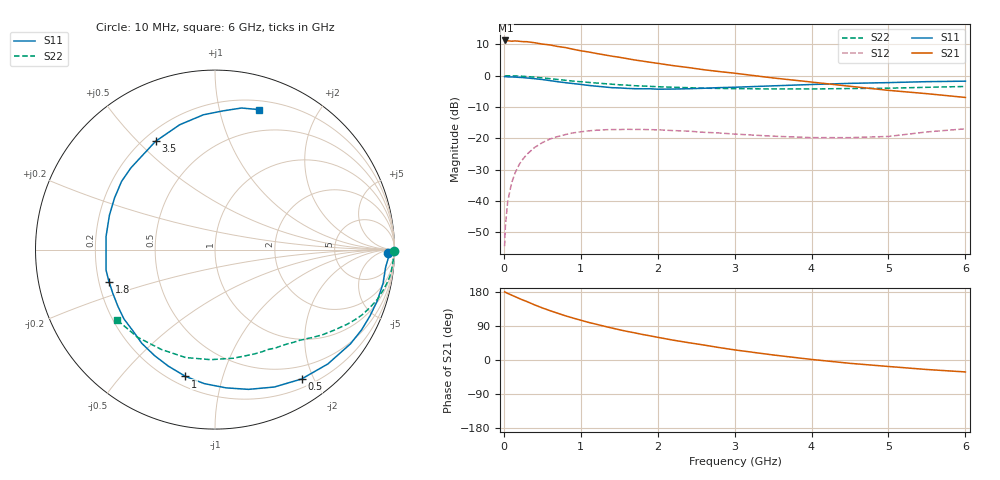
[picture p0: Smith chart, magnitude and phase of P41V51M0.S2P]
! SIEMENS Small Signal Semiconductors
! BFP182
! Si NPN RF Bipolar Junction Transistor in SOT143
! VCE = 1.5 V  IC = 1 mA
! Common Emitter S-Parameters:  March  1996
# GHz  S  MA  R  50
!  f  S11  S21  S12  S22
! GHz  MAG  ANG  MAG  ANG  MAG  ANG  MAG  ANG
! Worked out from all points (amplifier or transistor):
!   36 points, 10 MHz to 6 GHz, reference 50 ohm
!   highest |S21| = 11.2 dB at 20 MHz (marker M1)
!   |S21| within 3 dB of that: start of sweep to 939.9 MHz
!   unconditionally stable (mu >= 1): 2.569 GHz to end of sweep
!   at 250 MHz: K = 0.10, MSG = 18.7 dB, |S12| = -26.6 dB
!   at 1.4 GHz: K = 0.55, MSG = 11.7 dB, |S12| = -17.2 dB
!   at 6 GHz: K = 1.13, MAG = 2.8 dB, |S12| = -17.0 dB
!   S11 on the Smith chart (normalised r, x): 10 MHz: 42, -21; 500 MHz: 0.31, -1.83; 1 GHz: 0.26, -0.76; 1.8 GHz: 0.24, -0.14; 3.5 GHz: 0.25, +0.56; 6 GHz: 0.28, +1.32
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0.01  0.963 -1.1  3.57 179.5  0.0019 78.7  0.9985 -0.5
0.02  0.9681 -2.4  3.648 178.8  0.0039 88.4  0.9914 -0.9
0.05  0.9555 -6.0  3.609 175.7  0.0098 87.2  0.9969 -2.2
0.1  0.9551 -11.4  3.551 171.3  0.0193 81.6  0.9931 -4.4
0.15  0.9482 -17.5  3.587 166.9  0.0287 78.7  0.9901 -6.7
0.3  0.9195 -34.8  3.486 154.2  0.0556 68.6  0.9666 -13.1
0.4  0.8951 -45.4  3.354 145.4  0.0715 62.1  0.9465 -17.0
0.5  0.8674 -56.2  3.196 137.5  0.0853 55.4  0.9211 -20.6
0.6  0.8341 -66.6  3.094 130.2  0.0976 49.7  0.8968 -23.9
0.8  0.7726 -85.5  2.81 116.7  0.1149 39.6  0.8446 -29.6
1  0.7254 -103.1  2.497 104.9  0.1269 31.0  0.8001 -34.2
1.1  0.6995 -111.8  2.391 99.3  0.1315 27.2  0.781 -36.3
1.3  0.6627 -128.0  2.157 89.4  0.1369 20.3  0.7468 -40.2
1.5  0.6376 -142.8  1.968 79.9  0.1379 14.7  0.7158 -43.7
1.8  0.6172 -163.2  1.71 67.5  0.1386 8.2  0.6845 -48.3
2.2  0.6114 173.2  1.447 52.4  0.133 1.3  0.6526 -55.0
2.8  0.6445 143.9  1.163 32.8  0.1217 -4.7  0.6263 -65.6
3.5  0.6881 118.8  0.92 13.3  0.1082 -4.9  0.6138 -80.3
4  0.7229 105.8  0.791 1.5  0.1026 -0.8  0.6137 -92.3
4.5  0.754 94.9  0.677 -8.8  0.1025 3.4  0.6232 -105.2
5.5  0.8025 79.4  0.516 -25.1  0.1265 13.1  0.652 -131.7
6  0.8172 72.7  0.449 -31.5  0.1418 12.0  0.6724 -144.6
